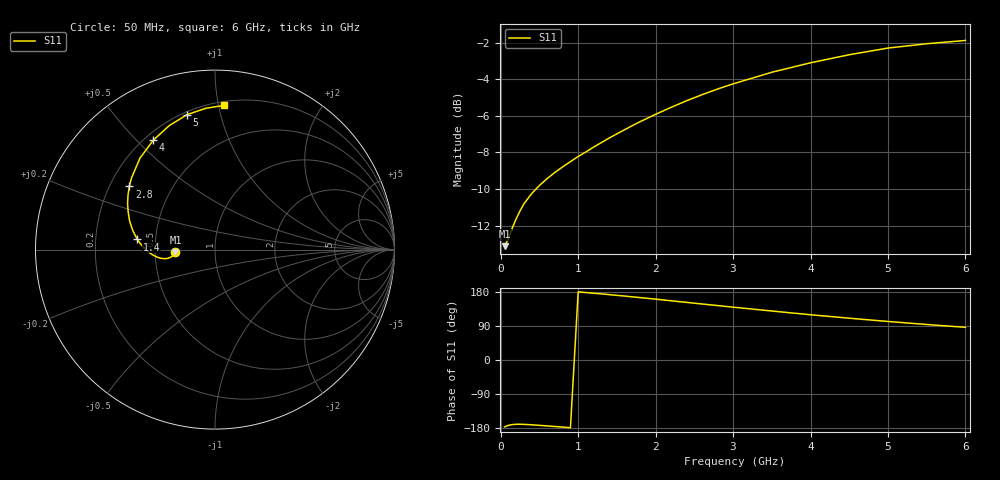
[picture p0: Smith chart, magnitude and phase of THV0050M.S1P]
! SIEMENS Discrete & RF Semiconductors
! BAS70
! Si Schottky Diode in SOT23
! IF = 50 mA
! S-Parameters:  February  1997
# GHz  S  MA  R  50
!  f  S11
! GHz  MAG  ANG
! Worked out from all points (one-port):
!   34 points, 50 MHz to 6 GHz, reference 50 ohm
!   lowest |S11| = -13.1 dB at 50 MHz (marker M1), VSWR 1.57, Z = 31.9 - j0.93 ohm
!   |S11| at or under -10 dB: start of sweep to 456 MHz
!   S11 on the Smith chart (normalised r, x): 50 MHz: 0.64, -0.02; 1.4 GHz: 0.39, +0.06; 2.8 GHz: 0.28, +0.31; 4 GHz: 0.23, +0.56; 5 GHz: 0.22, +0.79; 6 GHz: 0.23, +1.04
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0.05  0.2206 -176.4
0.1  0.2321 -172.4
0.15  0.2476 -170.5
0.2  0.2623 -169.6
0.25  0.2758 -169.5
0.3  0.2882 -169.9
0.4  0.3073 -171.0
0.5  0.3234 -172.5
0.6  0.3377 -174.0
0.8  0.3636 -177.0
1.1  0.3992 178.0
1.3  0.4235 174.5
1.4  0.4358 172.5
1.6  0.4592 168.7
1.8  0.4832 164.6
1.9  0.4944 162.7
2  0.506 160.6
2.2  0.5287 156.3
2.4  0.5512 152.1
2.6  0.5725 147.8
2.8  0.5934 143.6
3  0.6128 139.4
3.5  0.6594 129.3
4  0.6998 119.4
4.5  0.7362 110.3
5  0.7679 101.7
5.5  0.789 93.7
6  0.8055 86.3
